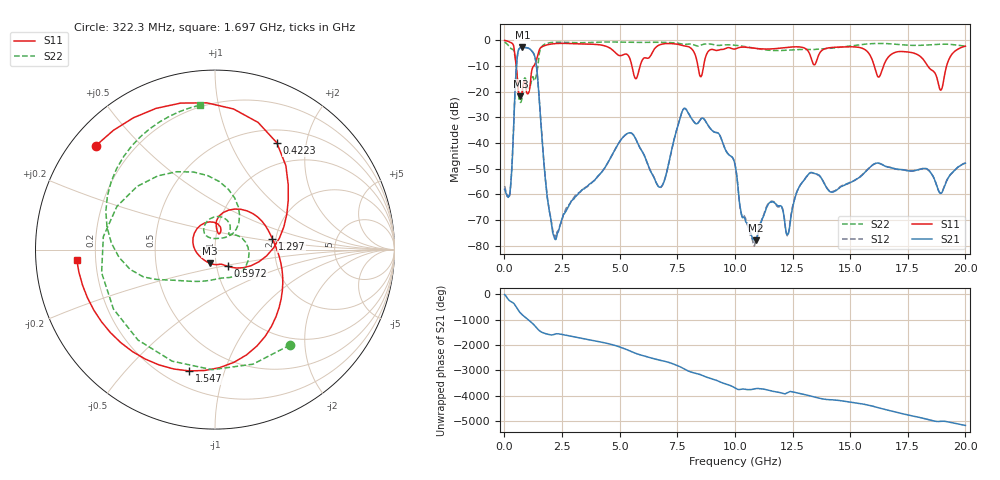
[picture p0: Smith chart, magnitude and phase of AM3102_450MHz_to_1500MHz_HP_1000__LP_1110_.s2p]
!Agilent Technologies,E8364B,MY43040894,A.07.50.67
!Agilent E8364B: A.07.50.67
!Date: Thursday, January 11, 2018 06:00:10
!Correction: S11(Full 2 Port(1,2))
!S21(Full 2 Port(1,2))
!S12(Full 2 Port(1,2))
!S22(Full 2 Port(1,2))
!S2P File: Measurements: S11, S21, S12, S22:
# Hz S  dB  R 50
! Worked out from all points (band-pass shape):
!   1601 points, 10 MHz to 20 GHz, reference 50 ohm
!   highest |S21| = -2.75 dB at 784.6 MHz (marker M1); lowest = -77.9 dB at 10.9 GHz (marker M2)
!   |S21| within 3 dB of the highest: 569.2 MHz to 1.3 GHz (730.5 MHz wide, 78.2 % of centre)
!   lowest |S11| = -21.8 dB at 697.2 MHz (marker M3), VSWR 1.18, Z = 46.5 - j7.05 ohm
!   |S11| at or under -10 dB: 513.1 MHz to 1.275 GHz (762.1 MHz wide, 85.2 % of centre); 16.05 GHz to 16.45 GHz (400.9 MHz wide, 2.47 % of centre); 18.37 GHz to 19.18 GHz (819.8 MHz wide, 4.37 % of centre)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
!   |S22| runs from -24.2 to -0.6 dB; largest |S21 - S12| = 0.0014
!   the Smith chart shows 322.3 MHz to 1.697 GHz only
!   S11 on the Smith chart (normalised r, x): 322.3 MHz: 0.07, +0.37; 422.3 MHz: 0.67, +1.52; 597.2 MHz: 1.13, -0.21; 1.297 GHz: 1.92, +0.26; 1.547 GHz: 0.30, -0.77; 1.697 GHz: 0.13, -0.04
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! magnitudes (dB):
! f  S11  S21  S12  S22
! 10 MHz  -0.1  -58.0  -56.8  -0.7
! 322.3 MHz  -1.1  -50.0  -50.0  -3.4
! 422.3 MHz  -3.3  -28.3  -28.4  -4.5
! 597.2 MHz  -18.6  -4.2  -4.2  -19.5
! 697.2 MHz  -21.8  -2.9  -2.9  -24.2
! 784.6 MHz  -19.2  -2.8  -2.8  -20.7
! 1.297 GHz  -9.8  -5.7  -5.7  -15.8
! 1.547 GHz  -3.2  -27.4  -27.4  -3.8
! 1.697 GHz  -2.2  -45.8  -45.7  -1.8
! 2.184 GHz  -1.3  -77.2  -76.1  -0.7
! 3.346 GHz  -1.4  -58.6  -58.5  -0.9
! 5.42 GHz  -6.6  -36.1  -36.1  -0.8
! 6.682 GHz  -2.0  -57.0  -57.0  -0.8
! 7.819 GHz  -2.2  -26.5  -26.5  -1.6
! 10.01 GHz  -3.4  -48.5  -48.4  -1.9
! 10.9 GHz  -3.2  -77.9  -78.4  -3.2
! 11.58 GHz  -3.4  -62.9  -62.7  -3.9
! 12.3 GHz  -2.7  -75.6  -76.0  -3.9
! 13.34 GHz  -7.9  -51.5  -51.6  -3.6
! 16.68 GHz  -6.3  -49.5  -49.4  -1.3
! 18.93 GHz  -19.4  -59.6  -59.4  -1.5
! 20 GHz  -2.3  -47.9  -47.8  -2.3
